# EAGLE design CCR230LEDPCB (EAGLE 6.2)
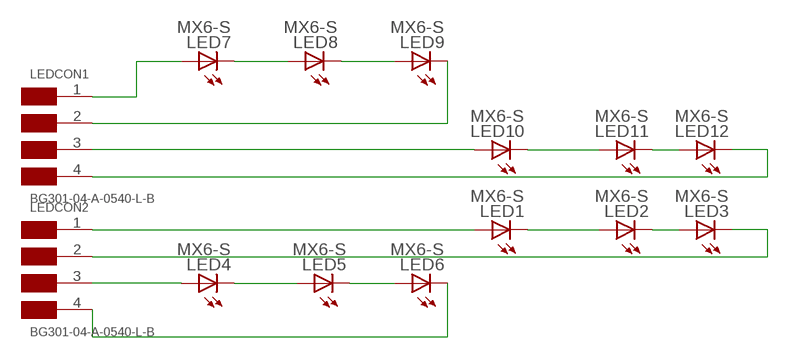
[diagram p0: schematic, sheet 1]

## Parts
LED1  MX6-S  [MX6-S]
LED2  MX6-S  [MX6-S]
LED3  MX6-S  [MX6-S]
LED4  MX6-S  [MX6-S]
LED5  MX6-S  [MX6-S]
LED6  MX6-S  [MX6-S]
LED7  MX6-S  [MX6-S]
LED8  MX6-S  [MX6-S]
LED9  MX6-S  [MX6-S]
LED10  MX6-S  [MX6-S]
LED11  MX6-S  [MX6-S]
LED12  MX6-S  [MX6-S]
LEDCON1  BG301-04-A-0540-L-B  [LEDCON_4_M]
LEDCON2  BG301-04-A-0540-L-B  [LEDCON_4_M]

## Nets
LED1: LED4.C LED5.A
LED2: LED5.C LED6.A
N$1: LED1.A LEDCON2.1
N$6: LED7.C LED8.A
N$7: LED8.C LED9.A
N$8: LED10.C LED11.A
N$10: LED3.C LEDCON2.2
N$11: LED4.A LEDCON2.3
N$12: LED6.C LEDCON2.4
N$13: LED7.A LEDCON1.1
N$14: LED9.C LEDCON1.2
N$15: LED10.A LEDCON1.3
QWFW: LED11.C LED12.A
RJ: LED12.C LEDCON1.4
RJT: LED1.C LED2.A
WGG: LED2.C LED3.A

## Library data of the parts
LED1-LED12 = CCR_120VAC_LIB:MX6-S
LEDCON1 LEDCON2 = CCR_120VAC_LIB:BG301-04-A-0540-L-B

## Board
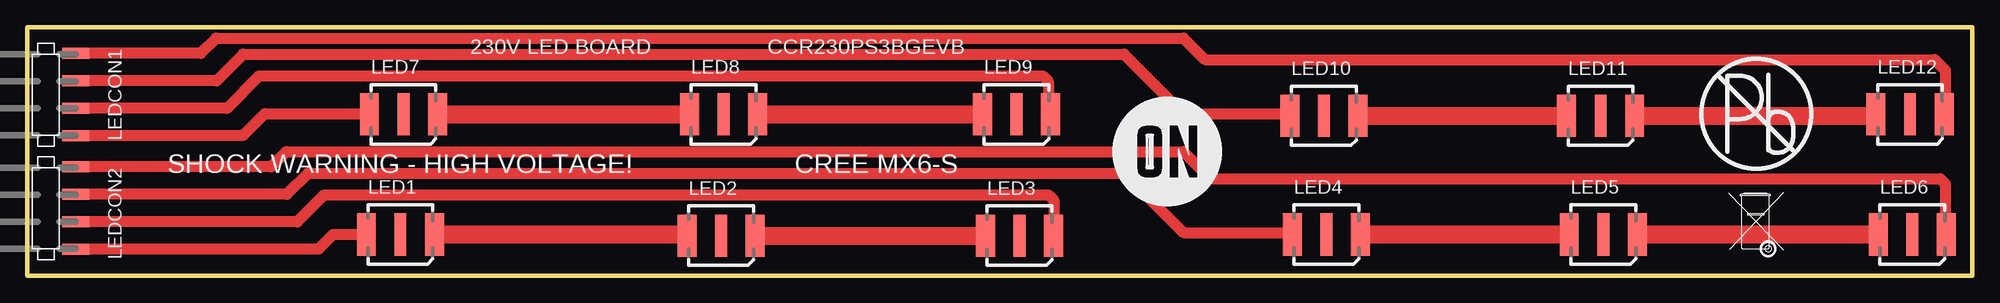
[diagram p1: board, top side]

Size 180 x 23 mm. Coordinates in mm from the lower left corner, seen from the top.
Outline: 0,0 0,23 180,23 180,0 0,0
Copper layers (1*16): Top 0.035mm / dielectric 1.5mm / Bottom 0.035mm
Design rules "default": minimum track width 10mil, minimum drill 24mil, track to track 8mil, track to pad 8mil, pad to pad 8mil, via to via 8mil, smd to smd 8mil, copper to edge 40mil, drill to drill 8mil, minimum pad ring 10mil, minimum via ring 8mil, stop-mask expansion 4mil, vias tented up to drill 0mil, thermal gap 10mil

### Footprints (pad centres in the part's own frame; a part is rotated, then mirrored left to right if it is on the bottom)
MX6-S = smd 1.75 x 3.9: A -3.15,0; C 3.15,0 | smd 1.1 x 3.9: P$1 0,0
LEDCON_4_M = smd 2.5 x 1: 1 0,2.54; 2 0,0; 3 0,-2.54; 4 0,-5.08

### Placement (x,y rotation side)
LED1  34.55,3.83 0 top
LED2  64.22,3.72 0 top
LED3  91.83,3.72 0 top
LED4  120.22,3.83 0 top
LED5  145.83,3.83 0 top
LED6  174.44,3.83 0 top
LED7  34.83,14.94 0 top
LED8  64.44,14.94 0 top
LED9  91.55,14.94 0 top
LED10  119.98,14.81 0 top
LED11  145.59,14.81 0 top
LED12  174.22,14.94 0 top
LEDCON1  4.5,15.5 180 top
LEDCON2  4.5,5 180 top
U$1  [ON1]  105.5,11.5 0 top
U$2  [PB]  160,15 0 top
U$3  [BIN1]  160,5 0 top

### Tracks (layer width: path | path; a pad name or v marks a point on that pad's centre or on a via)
LED1
  Top 1.676: LED4.C LED5.A
LED2
  Top 1.676: LED5.C LED6.A
N$1
  Top 1.016: LEDCON2.1 4.54,2.5 27,2.5 28.33,3.83 LED1.A
N$6
  Top 1.676: LED7.C LED8.A
N$7
  Top 1.676: LED8.C LED9.A
N$8
  Top 1.676: LED10.C LED11.A
N$10
  Top 1.016: LED3.C 95,3.74 95,7 94.5,7.5 27.5,7.5 25,5 LEDCON2.2
N$11
  Top 1.016: LED4.A 116.9,4 107,4 101.5,9.5 26,9.5 24.04,7.54 LEDCON2.3
N$12
  Top 1.016: LED6.C 177.5,3.92 177.5,8.5 177,9 109.5,9 107,11.5 24,11.5 22.58,10.08 LEDCON2.4
N$13
  Top 1.016: LED7.A 31.62,15 22,15 19.96,12.96 LEDCON1.1
N$14
  Top 1.016: LED9.C 94.5,15.14 94.5,18 94,18.5 21.5,18.5 18.5,15.5 LEDCON1.2
N$15
  Top 1.016: LED10.A 116.64,15 107,15 101.5,20.5 20,20.5 17.54,18.04 LEDCON1.3
QWFW
  Top 1.676: LED11.C 170.94,14.81 LED12.A
RJ
  Top 1.016: LED12.C 177.5,15.07 177.5,19 176.5,20 109,20 107,22 17.5,22 16.08,20.58 LEDCON1.4
RJT
  Top 1.676: LED1.C 60.96,3.83 LED2.A
WGG
  Top 1.676: LED2.C LED3.A

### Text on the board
tNames: 230V LED BOARD | CCR230PS3BGEVB | SHOCK WARNING - HIGH VOLTAGE! | CREE MX6-S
